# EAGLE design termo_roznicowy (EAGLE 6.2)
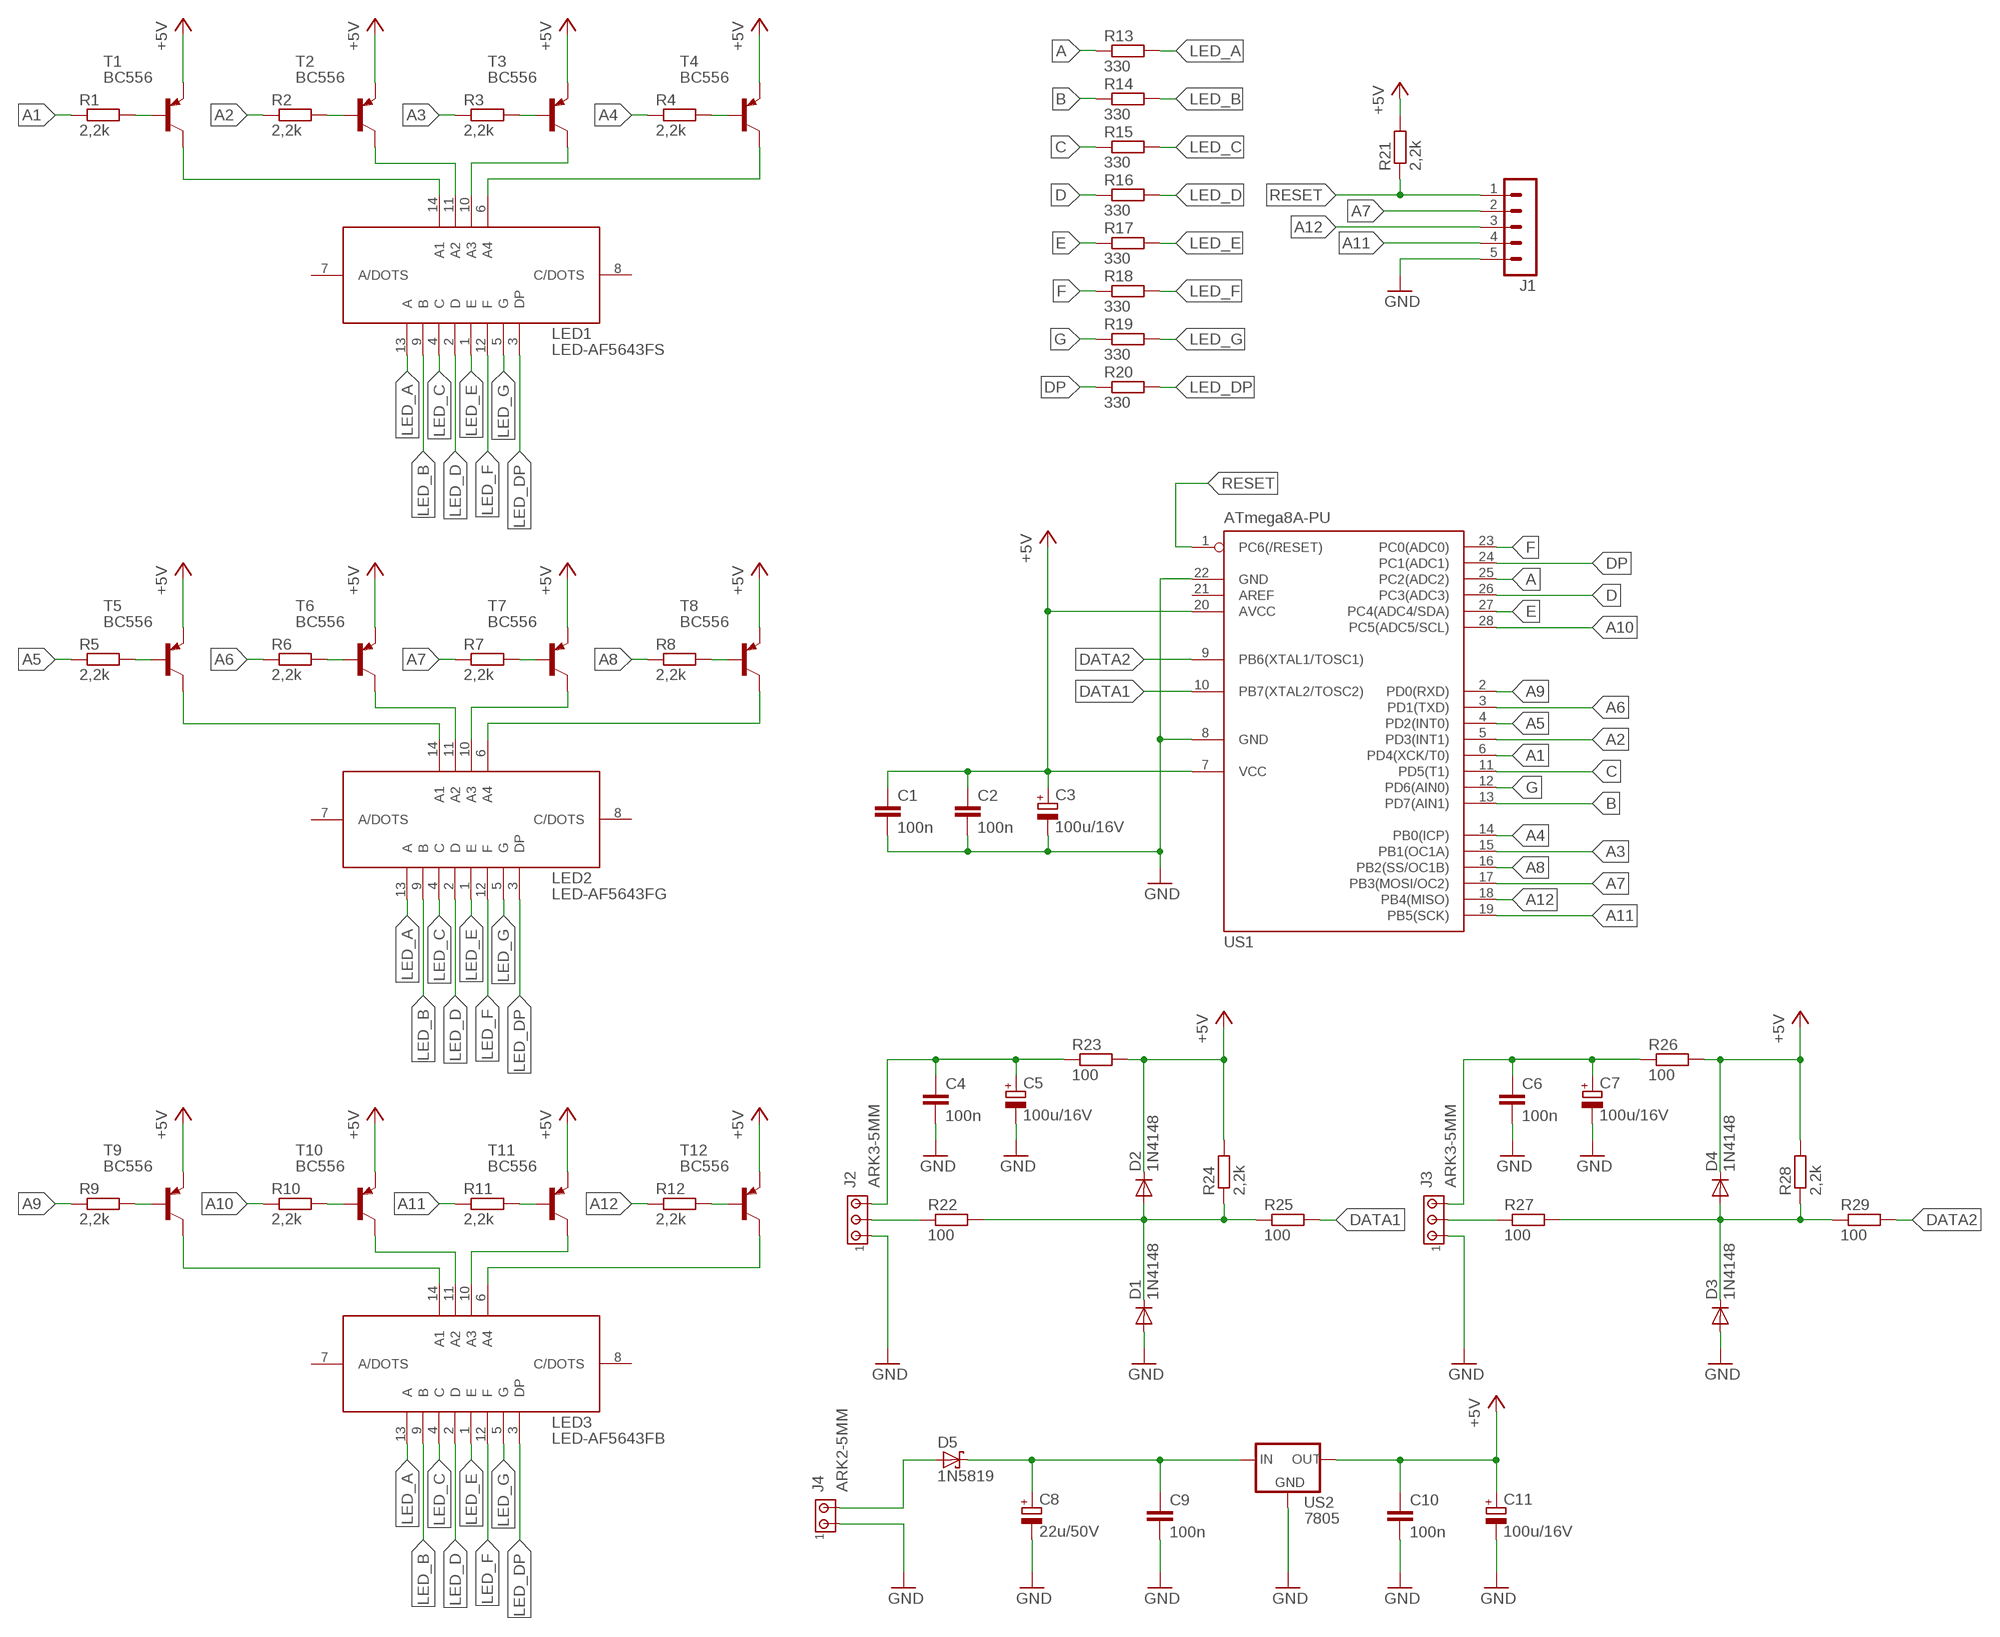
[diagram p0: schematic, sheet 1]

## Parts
C1  100n  C-EU050-025X075  [C050-025X075]
C2  100n  C-EU050-025X075  [C050-025X075]
C3  100u/16V  CPOL-EUE2.5-5  [E2,5-5]
C4  100n  C-EU050-025X075  [C050-025X075]
C5  100u/16V  CPOL-EUE2.5-5  [E2,5-5]
C6  100n  C-EU050-025X075  [C050-025X075]
C7  100u/16V  CPOL-EUE2.5-5  [E2,5-5]
C8  22u/50V  CPOL-EUE2.5-5  [E2,5-5]
C9  100n  C-EU050-025X075  [C050-025X075]
C10  100n  C-EU050-025X075  [C050-025X075]
C11  100u/16V  CPOL-EUE2.5-5  [E2,5-5]
D1  1N4148  BAT81  [DO34-7]
D2  1N4148  BAT81  [DO34-7]
D3  1N4148  BAT81  [DO34-7]
D4  1N4148  BAT81  [DO34-7]
D5  1N5819  1N5817-T  [DO41-7.6]
J1  MA05-1  [MA05-1]
J2  ARK3-5MM  [3PIN-5MM]
J3  ARK3-5MM  [3PIN-5MM]
J4  ARK2-5MM  [2PIN-5MM]
LED1  LED-AF5643FS  LED_DISP_AF5643FS  [LED_DISP_AF5643FS]
LED2  LED-AF5643FG  LED_DISP_AF5643FS  [LED_DISP_AF5643FS]
LED3  LED-AF5643FB  LED_DISP_AF5643FS  [LED_DISP_AF5643FS]
R1  2,2k  R-EU_0207/7  [0207/7]
R2  2,2k  R-EU_0207/7  [0207/7]
R3  2,2k  R-EU_0207/7  [0207/7]
R4  2,2k  R-EU_0207/7  [0207/7]
R5  2,2k  R-EU_0207/7  [0207/7]
R6  2,2k  R-EU_0207/7  [0207/7]
R7  2,2k  R-EU_0207/7  [0207/7]
R8  2,2k  R-EU_0207/7  [0207/7]
R9  2,2k  R-EU_0207/7  [0207/7]
R10  2,2k  R-EU_0207/7  [0207/7]
R11  2,2k  R-EU_0207/7  [0207/7]
R12  2,2k  R-EU_0207/7  [0207/7]
R13  330  R-EU_0207/7  [0207/7]
R14  330  R-EU_0207/7  [0207/7]
R15  330  R-EU_0207/7  [0207/7]
R16  330  R-EU_0207/7  [0207/7]
R17  330  R-EU_0207/7  [0207/7]
R18  330  R-EU_0207/7  [0207/7]
R19  330  R-EU_0207/7  [0207/7]
R20  330  R-EU_0207/7  [0207/7]
R21  2,2k  R-EU_0207/7  [0207/7]
R22  100  R-EU_0207/7  [0207/7]
R23  100  R-EU_0207/7  [0207/7]
R24  2,2k  R-EU_0207/7  [0207/7]
R25  100  R-EU_0207/7  [0207/7]
R26  100  R-EU_0207/7  [0207/7]
R27  100  R-EU_0207/7  [0207/7]
R28  2,2k  R-EU_0207/7  [0207/7]
R29  100  R-EU_0207/7  [0207/7]
T1  BC556  [TO92-EBC]
T2  BC556  [TO92-EBC]
T3  BC556  [TO92-EBC]
T4  BC556  [TO92-EBC]
T5  BC556  [TO92-EBC]
T6  BC556  [TO92-EBC]
T7  BC556  [TO92-EBC]
T8  BC556  [TO92-EBC]
T9  BC556  [TO92-EBC]
T10  BC556  [TO92-EBC]
T11  BC556  [TO92-EBC]
T12  BC556  [TO92-EBC]
US1  ATmega8A-PU  MEGA8-P  [DIL28-3]
US2  7805  78XXS  [78XXS]

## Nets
+5V: C1.1 C2.1 C3.+ C10.1 C11.+ D2.C D4.C R21.2 R23.2 R24.2 R26.2 R28.2 T1.E T2.E T3.E T4.E T5.E T6.E T7.E T8.E T9.E T10.E T11.E T12.E US1.7(VCC) US1.20(AVCC) US2.OUT
A: R13.1 US1.25(PC2(ADC2))
A1: R1.1 US1.6(PD4(XCK/T0))
A2: R2.1 US1.5(PD3(INT1))
A3: R3.1 US1.15(PB1(OC1A))
A4: R4.1 US1.14(PB0(ICP))
A5: R5.1 US1.4(PD2(INT0))
A6: R6.1 US1.3(PD1(TXD))
A7: J1.2 R7.1 US1.17(PB3(MOSI/OC2))
A8: R8.1 US1.16(PB2(SS/OC1B))
A9: R9.1 US1.2(PD0(RXD))
A10: R10.1 US1.28(PC5(ADC5/SCL))
A11: J1.4 R11.1 US1.19(PB5(SCK))
A12: J1.3 R12.1 US1.18(PB4(MISO))
B: R14.1 US1.13(PD7(AIN1))
C: R15.1 US1.11(PD5(T1))
D: R16.1 US1.26(PC3(ADC3))
DATA1: R25.2 US1.10(PB7(XTAL2/TOSC2))
DATA2: R29.2 US1.9(PB6(XTAL1/TOSC1))
DP: R20.1 US1.24(PC1(ADC1))
E: R17.1 US1.27(PC4(ADC4/SDA))
F: R18.1 US1.23(PC0(ADC0))
G: R19.1 US1.12(PD6(AIN0))
GND: C1.2 C2.2 C3.- C4.2 C5.- C6.2 C7.- C8.- C9.2 C10.2 C11.- D1.A D3.A J1.5 J2.P$1 J3.P$1 J4.P$1 US1.8(GND) US1.22(GND) US2.GND
LED_A: LED1.13(A) LED2.13(A) LED3.13(A) R13.2
LED_B: LED1.9(B) LED2.9(B) LED3.9(B) R14.2
LED_C: LED1.4(C) LED2.4(C) LED3.4(C) R15.2
LED_D: LED1.2(D) LED2.2(D) LED3.2(D) R16.2
LED_DP: LED1.3(DP) LED2.3(DP) LED3.3(DP) R20.2
LED_E: LED1.1(E) LED2.1(E) LED3.1(E) R17.2
LED_F: LED1.12(F) LED2.12(F) LED3.12(F) R18.2
LED_G: LED1.5(G) LED2.5(G) LED3.5(G) R19.2
N$1: R1.2 T1.B
N$2: R2.2 T2.B
N$3: R3.2 T3.B
N$4: R4.2 T4.B
N$5: LED1.14(A1) T1.C
N$6: LED1.11(A2) T2.C
N$7: LED1.10(A3) T3.C
N$8: LED1.6(A4) T4.C
N$9: R5.2 T5.B
N$10: R6.2 T6.B
N$11: R7.2 T7.B
N$12: R8.2 T8.B
N$13: LED2.14(A1) T5.C
N$14: LED2.11(A2) T6.C
N$15: LED2.10(A3) T7.C
N$16: LED2.6(A4) T8.C
N$17: R9.2 T9.B
N$18: R10.2 T10.B
N$19: R11.2 T11.B
N$20: R12.2 T12.B
N$21: LED3.14(A1) T9.C
N$22: LED3.11(A2) T10.C
N$23: LED3.10(A3) T11.C
N$24: LED3.6(A4) T12.C
N$25: C6.1 C7.+ J3.P$3 R26.1
N$26: D5.A J4.P$2
N$27: C8.+ C9.1 D5.C US2.IN
N$28: C4.1 C5.+ J2.P$3 R23.1
N$29: D1.C D2.A R22.2 R24.1 R25.1
N$30: J2.P$2 R22.1
N$31: J3.P$2 R27.1
N$32: D3.C D4.A R27.2 R28.1 R29.1
RESET: J1.1 R21.1 US1.1(PC6(/RESET))
Unconnected: LED1.7(A/DOTS) LED1.8(C/DOTS) LED2.7(A/DOTS) LED2.8(C/DOTS) LED3.7(A/DOTS) LED3.8(C/DOTS) US1.21(AREF)

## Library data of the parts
C1 C2 C4 C6 C9 C10 = rcl:C-EU: CAPACITOR, European symbol
C3 C5 C7 C8 C11 = rcl:CPOL-EU: POLARIZED CAPACITOR, European symbol
D1-D4 = diode:BAT81: DIODE
D5 = diode:1N581*: 1.0A SCHOTTKY BARRIER RECTIFIER
J1 = zlacza_futrzak:MA05-1: PIN HEADER; OC_FARNELL: unknown; OC_NEWARK: unknown
J2 J3 = zlacza_futrzak:ARK3: ARK 3 Raster 5mm i 3,5mm
J4 = zlacza_futrzak:ARK2: ARK 2
LED1-LED3 = inne_futrzak:LED_DISP_AF5643FS
R1-R29 = rcl:R-EU_: RESISTOR, European symbol
T1-T12 = transistor-pnp:BC556*: PNP Transistror
US1 = atmel:MEGA8-P: MICROCONTROLLER 8 Kbytes FLASH, 1 kbytes SRAM, 512 bytes EEPROM, USART, 4-channel 10 bit ADC, 2-channel 8 bit ADC Pin compatible with Atmega48, ATMega88, ATMega168 Source: avr.lbr; OC_FARNELL: unknown; OC_NEWARK: unknown
US2 = v-reg:78XXS: VOLTAGE REGULATOR

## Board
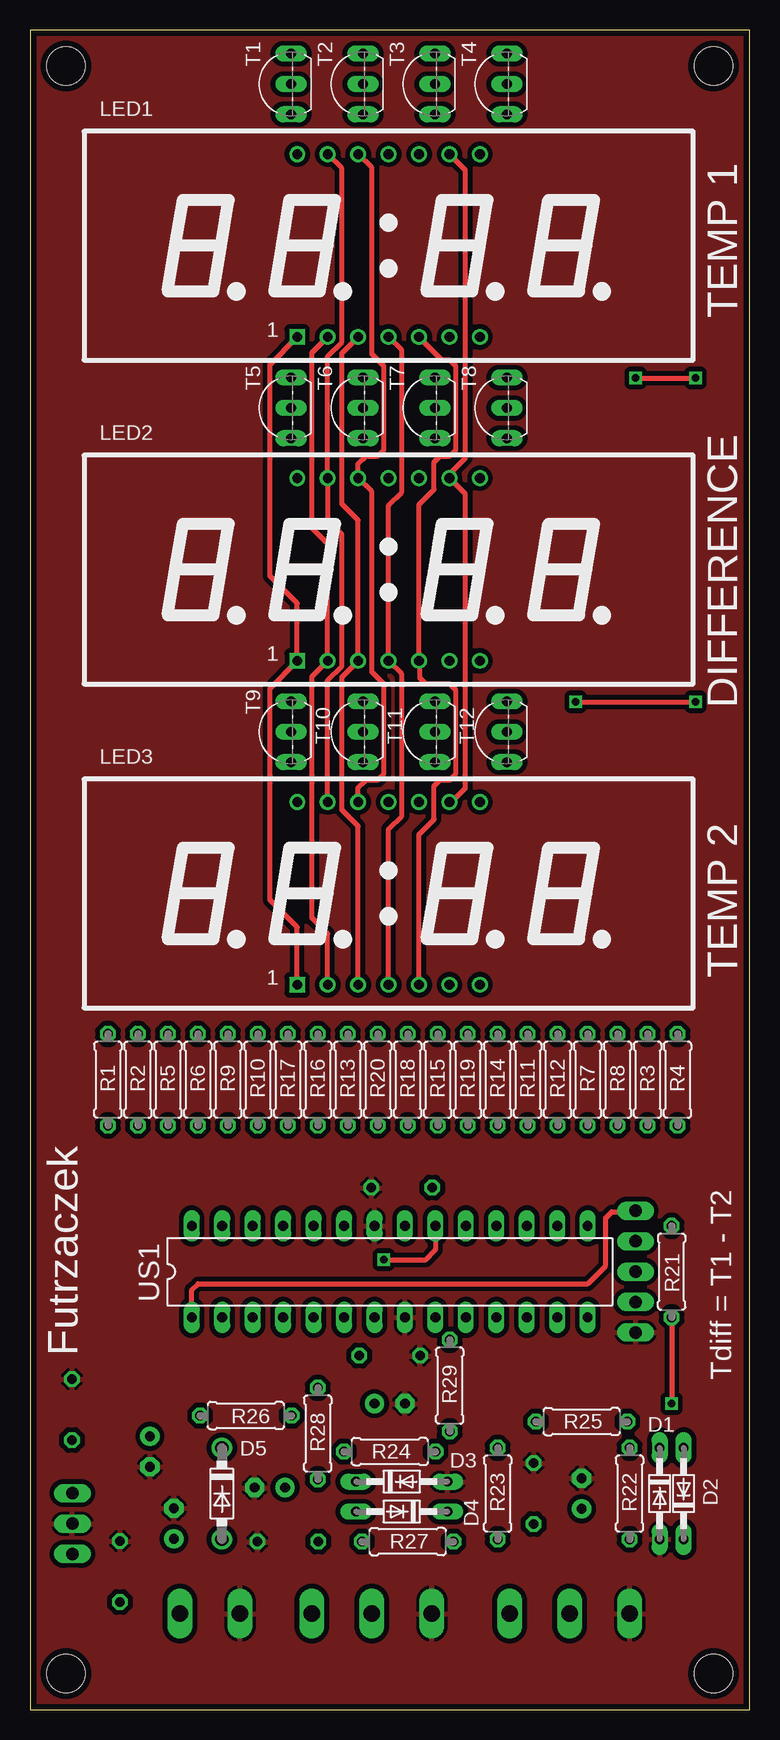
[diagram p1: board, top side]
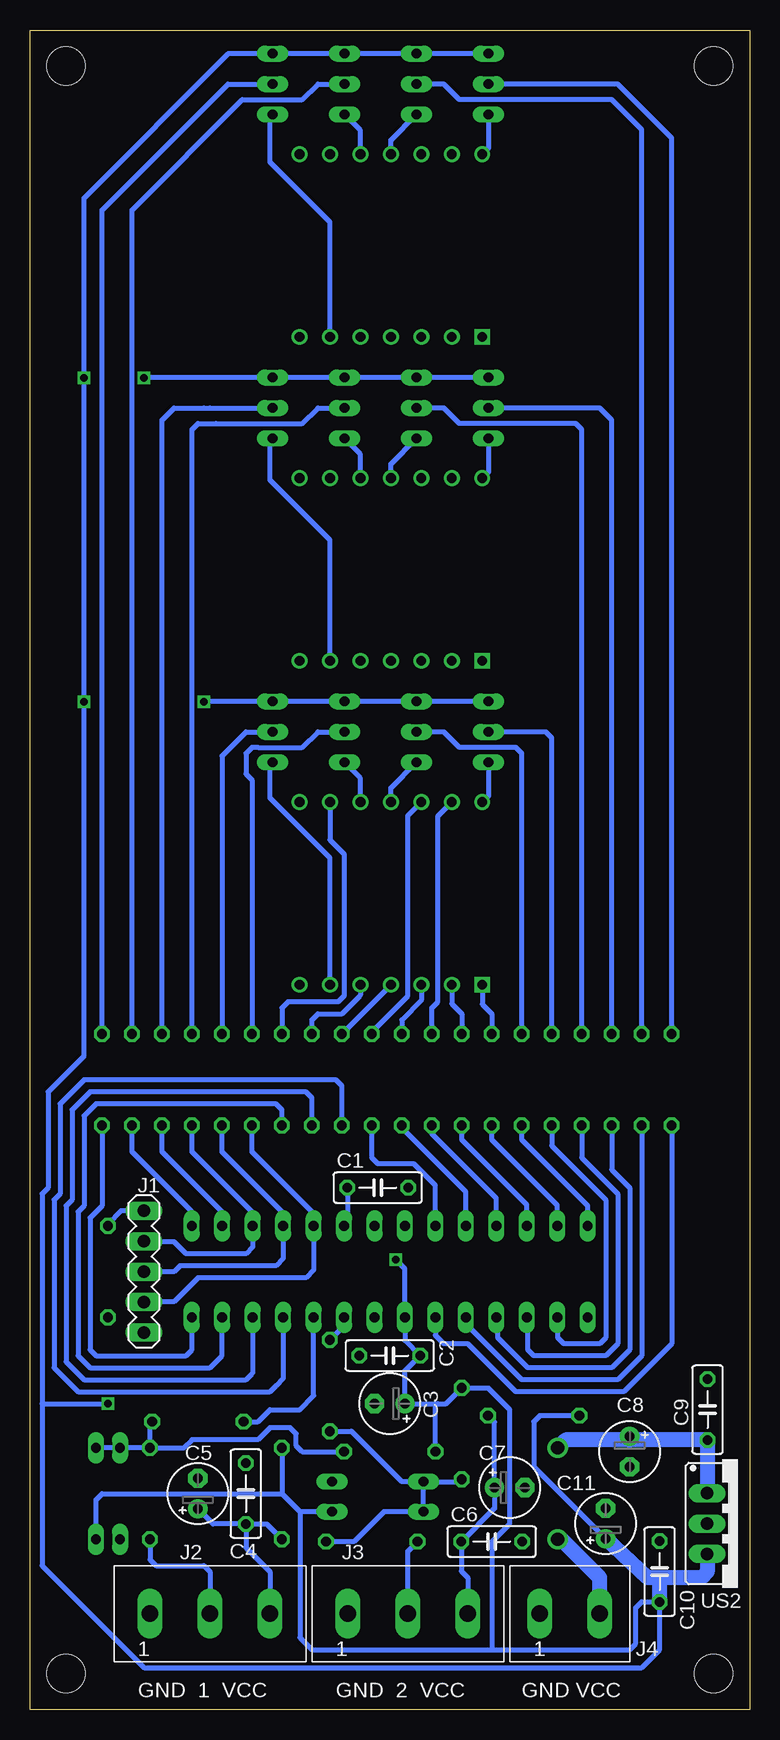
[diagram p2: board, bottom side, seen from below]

Size 60 x 140 mm. Coordinates in mm from the lower left corner, seen from the top.
Outline: 0,0 60,0 60,140 0,140 0,0
Copper layers (1*16): Top 0.035mm / dielectric 1.5mm / Bottom 0.035mm
Design rules: minimum track width 10mil, minimum drill 23mil, track to track 8mil, track to pad 8mil, pad to pad 8mil, via to via 8mil, smd to smd 8mil, copper to edge 20mil, drill to drill 8mil, minimum pad ring 10mil, minimum via ring 8mil, stop-mask expansion 4mil, vias tented up to drill 0mil, thermal gap 10mil
Holes 3.2 mm at 3,137 57,137 3,3 57,3

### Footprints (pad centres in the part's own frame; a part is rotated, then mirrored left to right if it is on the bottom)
C050-025X075 = drill 0.813 octagon: 1 -2.54,0; 2 2.54,0
E2,5-5 = drill 0.813 pad 1.6: + -1.27,0 | drill 0.813 pad 1.6 octagon: - 1.27,0
DO34-7 = drill 0.813 long: A 3.81,0; C -3.81,0
DO41-7.6 = drill 1.1 pad 1.7: A 3.81,0; C -3.81,0
MA05-1 = drill 1.016 long: 1 -5.08,0; 2 -2.54,0; 3 0,0; 4 2.54,0; 5 5.08,0
3PIN-5MM = drill 1.4 long: P$1 -5,0; P$2 0,0; P$3 5,0
2PIN-5MM = drill 1.4 long: P$1 -2.5,0; P$2 2.5,0
LED_DISP_AF5643FS = drill 0.8 square: 1 17.78,1.905 | drill 0.8: 2 20.32,1.905; 3 22.86,1.905; 4 25.4,1.905; 5 27.94,1.905; 6 30.48,1.905; 7 33.02,1.905; 8 33.02,17.145; 9 30.48,17.145; 10 27.94,17.145; 11 25.4,17.145; 12 22.86,17.145; 13 20.32,17.145; 14 17.78,17.145
0207/7 = drill 0.813 octagon: 1 -3.81,0; 2 3.81,0
TO92-EBC = drill 0.813 long: B 0,-1.27; C -2.54,-1.27; E 2.54,-1.27
DIL28-3 = drill 0.813 long: 1 -16.51,-3.81; 2 -13.97,-3.81; 3 -11.43,-3.81; 4 -8.89,-3.81; 5 -6.35,-3.81; 6 -3.81,-3.81; 7 -1.27,-3.81; 8 1.27,-3.81; 9 3.81,-3.81; 10 6.35,-3.81; 11 8.89,-3.81; 12 11.43,-3.81; 13 13.97,-3.81; 14 16.51,-3.81; 15 16.51,3.81; 16 13.97,3.81; 17 11.43,3.81; 18 8.89,3.81; 19 6.35,3.81; 20 3.81,3.81; 21 1.27,3.81; 22 -1.27,3.81; 23 -3.81,3.81; 24 -6.35,3.81; 25 -8.89,3.81; 26 -11.43,3.81; 27 -13.97,3.81; 28 -16.51,3.81
78XXS = drill 1.016 long: GND 0,-2.54; IN -2.54,-2.54; OUT 2.54,-2.54

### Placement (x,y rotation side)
C1  31,43.5 0 bottom
C2  30,29.5 180 bottom
C3  30,25.5 180 bottom
C4  42,18 90 bottom
C5  46,18 90 bottom
C6  21.5,14 0 bottom
C7  20,18.5 0 bottom
C8  10,21.5 270 bottom
C9  3.5,25 90 bottom
C10  7.5,11.5 90 bottom
C11  12,15.5 90 bottom
D1  52.5,18 270 top
D2  54.5,18 90 top
D3  31,19 0 top
D4  31,16.5 180 top
D5  16,18 270 top
J1  50.5,36.5 270 bottom
J2  45,8 0 bottom
J3  28.5,8 0 bottom
J4  15,8 0 bottom
LED1  4.5,112.5 0 top
LED2  4.5,85.5 0 top
LED3  4.5,58.5 0 top
R1  6.5,52.5 90 top
R2  9,52.5 90 top
R3  51.5,52.5 90 top
R4  54,52.5 90 top
R5  11.5,52.5 90 top
R6  14,52.5 90 top
R7  46.5,52.5 90 top
R8  49,52.5 90 top
R9  16.5,52.5 90 top
R10  19,52.5 90 top
R11  41.5,52.5 90 top
R12  44,52.5 90 top
R13  26.5,52.5 90 top
R14  39,52.5 90 top
R15  34,52.5 90 top
R16  24,52.5 90 top
R17  21.5,52.5 90 top
R18  31.5,52.5 90 top
R19  36.5,52.5 90 top
R20  29,52.5 90 top
R21  53.5,36.5 270 top
R22  50,18 90 top
R23  39,18 90 top
R24  30,21.5 180 top
R25  46,24 180 top
R26  18,24.5 180 top
R27  31.5,14 0 top
R28  24,23 90 top
R29  35,27 90 top
T1  20.5,135.5 90 top
T2  26.5,135.5 90 top
T3  32.5,135.5 90 top
T4  38.5,135.5 90 top
T5  20.5,108.5 90 top
T6  26.5,108.5 90 top
T7  32.5,108.5 90 top
T8  38.5,108.5 90 top
T9  20.5,81.5 90 top
T10  26.5,81.5 90 top
T11  32.5,81.5 90 top
T12  38.5,81.5 90 top
US1  30,36.5 0 top
US2  1,15.5 270 bottom

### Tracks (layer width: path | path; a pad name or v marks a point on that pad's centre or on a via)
+5V  (via drill 0.6)
  Top 0.406: v45.5,84 v55.5,84 | v50.5,111 v55.5,111 | v29.5,37.5 33,37.5 33.81,38.31 US1.20 | R21.2 v53.5,25.5
  Bottom 0.406: T9.E T10.E T11.E T12.E 45.46,84.04 v45.5,84 | T5.E T6.E T7.E T8.E 50.46,111.04 v50.5,111 | T1.E T2.E T3.E T4.E 43.46,138.04 55.5,126 v55.5,111 v55.5,84 55.5,54.5 58.5,51.5 58.5,43.5 59,43 59,25.5 | 59,25.5 v53.5,25.5 | 59,25.5 59,12 50.5,3.5 9,3.5 7.5,5 C10.1 7.54,9 9,9 9.5,8.5 9.5,5.5 10,5 21.5,5 | C1.1 33.54,40.58 US1.20 | v29.5,37.5 28.73,36.73 US1.7 28.73,30.77 C2.1 28.73,28.23 C3.+ 26,25.5 | R23.2 39,18 | D2.C 54.5,17.5 54,18 39,18 | 21.5,5 21.5,14 20,15.5 20,25 21.81,26.81 R28.2 25.31,25.5 26,25.5 | R26.2 17.5,24.5 18,24 18,20.23 C11.+ | R24.2 26.19,25.31 26,25.5 | 39,18 37.5,16.5 | 37.5,16.5 37.5,6 36.5,5 21.5,5 | D4.C 37.5,16.5
  Bottom 1.27: US2.OUT 3.54,11.46 4,11 7.5,11 | 7.5,11 8.52,11 C11.+ | C10.1 7.5,11
A
  Bottom 0.406: US1.25 21.11,42.61 26.5,48 R13.1
A1
  Bottom 0.406: R1.1 6.5,30.5 10.5,26.5 19.5,26.5 23.5,30.5 25.5,30.5 26.19,31.19 US1.6
A2
  Bottom 0.406: R2.1 9,29.5 11,27.5 19,27.5 23.5,32 23.5,32.54 US1.5
A3
  Bottom 0.406: US1.15 46.51,41.51 51.5,46.5 R3.1
A4
  Bottom 0.406: R4.1 54,42 55,41 55,30 54.5,29.5 47,29.5 46.5,30 US1.14
A5
  Bottom 0.406: R5.1 11.5,45 10,43.5 10,30 11.5,28.5 18.5,28.5 21,31 21,32.58 US1.4
A6
  Bottom 0.406: R6.1 14,46 11,43 11,30.5 12,29.5 18,29.5 18.5,30 18.5,32.62 US1.3
A7
  Bottom 0.406: R7.1 46.5,46.5 41.43,41.43 US1.17 41.43,38.57 42,38 47,38 48,39 50.46,39 J1.2
A8
  Bottom 0.406: US1.16 43.97,41.47 49,46.5 R8.1
A9
  Bottom 0.406: R9.1 16.5,47 12,42.5 12,31 12.5,30.5 15.5,30.5 16,31 16,32.66 US1.2
A10
  Bottom 0.406: US1.28 13.49,41.99 19,47.5 R10.1
A11
  Bottom 0.406: R11.1 41.5,46.5 36.35,41.35 US1.19 36.35,36.65 37,36 46,36 48,34 50.46,34 J1.4
A12
  Bottom 0.406: R12.1 44,46.5 38.89,41.39 US1.18 38.89,37.61 39.5,37 47.5,37 48,36.5 50,36.5 J1.3
B
  Bottom 0.406: R14.1 39,50 39.5,50.5 54.5,50.5 55,50 55.5,49.5 55.5,42 56,41.5 56,29.5 55,28.5 45,28.5 44,29.5 44,32.66 US1.13
C
  Bottom 0.406: R15.1 34,52 34.5,52.5 55.5,52.5 57.5,50.5 57.5,43 58,42.5 58,28.5 56,26.5 40,26.5 39.5,27 38.89,27.61 US1.11
D
  Bottom 0.406: US1.26 18.57,42.07 24,47.5 R16.1
DATA1
  Bottom 0.406: R25.2 41,24 40,25 37.5,25 36.35,26.15 US1.10
DATA2
  Bottom 0.406: US1.9 33.81,32 R29.2
DP
  Bottom 0.406: US1.24 23.65,43.15 26.5,46 29,48.5 R20.1
E
  Bottom 0.406: US1.27 16.03,42.03 21.5,47.5 R17.1
F
  Bottom 0.406: US1.23 26.19,43.69 27.5,45 28,45.5 31,45.5 31.5,46 R18.1
G
  Bottom 0.406: R19.1 36.5,51 37,51.5 55,51.5 56.5,50 56.5,42.5 57,42 57,29 55.5,27.5 42,27.5 41.5,28 41.43,28.07 US1.12
GND
  pour Top (isolate 0.406): 0,0 60,0 60,140 0,140
LED_A
  Top 0.406: LED3.13 24.82,85.82 26,87 26,97.97 24.82,99.14 LED2.13 24.82,112.82 26,114 26,128.47 LED1.13
  Bottom 0.406: R13.2 26.5,58.5 26,59 26,74.47 LED3.13
LED_B
  Top 0.406: LED3.9 35.15,75.64 36.3,76.8 36.3,101.33 LED2.9 34.98,102.98 36.3,104.3 36.3,128.32 LED1.9
  Bottom 0.406: LED3.9 34.98,72.48 33.8,71.3 33.8,59.5 34.3,59 38.5,59 39,58.5 R14.2
LED_C
  Top 0.406: LED3.4 29.9,73.4 31,74.5 31,86.31 LED2.4 29.9,100.4 31,101.5 31,113.31 LED1.4
  Bottom 0.406: R15.2 LED3.4
LED_D
  Top 0.406: LED3.2 24.82,64.68 23.5,66 23.5,86.08 LED2.2 24.82,97.18 23.5,98.5 23.5,113.08 LED1.2
  Bottom 0.406: LED3.2 24.82,58.82 24,58 R16.2
LED_DP
  Top 0.406: LED3.3 27.36,73.64 26,75 26,85.5 26,86.05 LED2.3 27.36,99.14 27,99.5 26,100.5 26,113.05 LED1.3
  Bottom 0.406: LED3.3 27.36,59.14 29,57.5 R20.2
LED_E
  Top 0.406: LED3.1 22.28,65.22 20,67.5 20,85.12 LED2.1 22.28,92.22 20,94.5 20,112.12 LED1.1
  Bottom 0.406: LED3.1 22.28,58.78 21.5,58 R17.2
LED_F
  Top 0.406: LED3.12 27.36,76.86 28,77.5 29,77.5 29.5,78 29.5,85.5 28.5,86.5 28.5,101.5 LED2.12 27.36,103.86 28,104.5 29,104.5 29.5,105 29.5,112 28.5,113 28.5,128.5 LED1.12
  Bottom 0.406: R18.2 31.5,56.5 28.5,59.5 28.5,74.5 LED3.12
LED_G
  Top 0.406: LED3.5 32.44,72.94 33.7,74.2 33.7,77 34.2,77.5 35,77.5 35.5,78 35.5,85 35,85.5 33,85.5 32.5,86 32.5,87.34 LED2.5 32.44,100.44 33.7,101.7 33.7,104 34.2,104.5 35,104.5 35.5,105 35.5,112 35,112.5 34.34,112.5 LED1.5
  Bottom 0.406: R19.2 36.5,57.5 36,58 34,58 32.5,59.5 32.44,59.56 LED3.5
N$1
  Bottom 0.406: R1.2 6.5,131 11,135.5 T1.B
N$2
  Bottom 0.406: R2.2 9,131.7 11.5,134.2 24.2,134.2 25.5,135.5 T2.B
N$3
  Bottom 0.406: R3.2 51.5,125 42.3,134.2 37.3,134.2 36,135.5 T3.B
N$4
  Bottom 0.406: R4.2 54,125 43.5,135.5 T4.B
N$5
  Bottom 0.406: T1.C 21.77,130.16 LED1.14
N$6
  Bottom 0.406: LED1.11 29.9,130.83 T2.C
N$7
  Bottom 0.406: LED1.10 32.44,131.63 T3.C
N$8
  Bottom 0.406: LED1.6 34.98,123.98 40,129 40,132.73 T4.C
N$9
  Bottom 0.406: R5.2 11.5,107.5 12.5,108.5 T5.B
N$10
  Bottom 0.406: R6.2 14,106.7 14.5,107.2 24.2,107.2 25.5,108.5 T6.B
N$11
  Bottom 0.406: T7.B 36,108.5 37.3,107.2 44.5,107.2 46,107.2 46.5,106.7 R7.2
N$12
  Bottom 0.406: 45.5,108.5 45,108.5 | 45,108.5 T8.B | R8.2 49,107.5 48,108.5 45,108.5
N$13
  Bottom 0.406: T5.C 21.77,103.16 LED2.14
N$14
  Bottom 0.406: LED2.11 29.9,103.83 T6.C
N$15
  Bottom 0.406: LED2.10 32.44,104.63 T7.C
N$16
  Bottom 0.406: LED2.6 34.98,97.48 40,102.5 40,105.73 T8.C
N$17
  Bottom 0.406: R9.2 16.5,81 17,81.5 T9.B
N$18
  Bottom 0.406: R10.2 19,79.7 19.5,80.2 24.2,80.2 25.5,81.5 T10.B
N$19
  Bottom 0.406: T11.B 36,81.5 37.3,80.2 41,80.2 41.5,80.2 42,79.7 42,78 41.5,77.5 R11.2
N$20
  Bottom 0.406: T12.B 42,81.5 43,80.5 44,79.5 R12.2
N$21
  Bottom 0.406: T9.C 21.77,76.16 LED3.14
N$22
  Bottom 0.406: LED3.11 29.9,76.83 T10.C
N$23
  Bottom 0.406: LED3.10 32.44,77.63 T11.C
N$24
  Bottom 0.406: LED3.6 34.98,70.98 40,76 40,78.73 T12.C
N$25
  Bottom 0.406: R26.1 21.27,23.96 C7.+ 21.27,16.77 C6.1 24.04,11.54 23.5,11 J3.P$3
N$26
  Bottom 1.27: J4.P$2 12.5,11 15.69,14.19 D5.A
N$27
  Bottom 1.27: US2.IN 3.5,18.04 C9.1 10,22.46 | 10,22.46 15.35,22.46 D5.C | C8.+ 10,22.46
N$28
  Bottom 0.406: C4.1 40.27,15.46 R23.1 | C4.1 42,13.5 40,11.5 J2.P$3 | C4.1 44.73,15.46 C5.+
N$29
  Bottom 0.406: 34,21.5 R24.1 37.3,21.5 37.8,22 37.8,23 38.3,23.5 40,23.5 41,22.5 46.5,22.5 47.19,21.81 R22.2 | R22.2 50,23.81 R25.1 | R22.2 D1.C D2.A
N$30
  Bottom 0.406: R22.1 50,12.5 49.5,12 45.5,12 45,11.5 J2.P$2
N$31
  Bottom 0.406: J3.P$2 28.5,13.19 R27.1
N$32
  Bottom 0.406: R27.2 33,14 30.5,16.5 D4.A D3.C | D3.C 24.19,19 R28.1 | D3.C 29,19 33.19,23.19 R29.1
RESET
  Top 0.406: US1.1 13.49,34.99 14,35.5 46.5,35.5 48,37 48,41 48.5,41.5 50.42,41.5 J1.1
  Bottom 0.406: J1.1 52.42,41.58 53.5,40.5 R21.1

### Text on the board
tPlace: TEMP 1 | DIFFERENCE | TEMP 2 | Futrzaczek | Tdiff = T1 - T2
bPlace: GND VCC | GND 2 VCC | GND 1 VCC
